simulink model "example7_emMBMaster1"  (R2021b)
settings: Solver=FixedStepAuto  StartTime=0  StopTime=inf  FixedStep=0.5  RelTol=1e-3  EnableMultiTasking=on
undefined symbols (not defined in the file or in its folder): based, classic, Coils, Discretes, dsPic33, InputsReg, MCC, Microchip, PIC24, Read
libraries: emMBMastedLib x8, embeddedCreatorLib x1

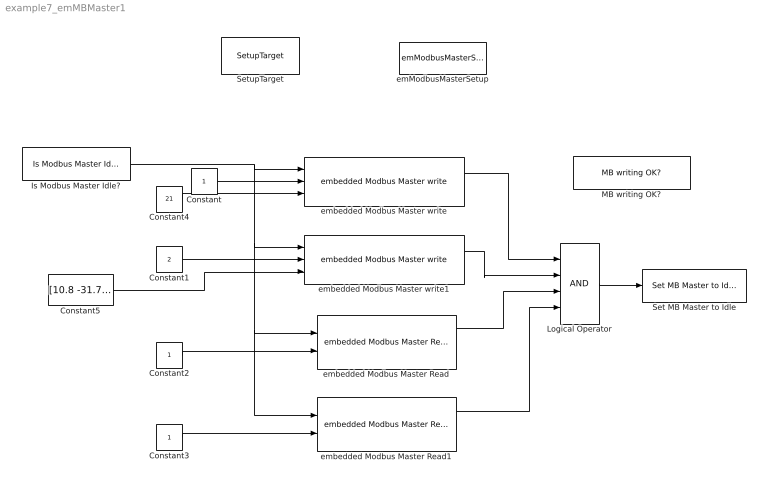
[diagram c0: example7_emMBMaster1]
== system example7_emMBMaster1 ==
  Constant : Constant  OutDataTypeStr=uint16
  Constant1 : Constant  Value=2  OutDataTypeStr=uint16
  Constant2 : Constant  OutDataTypeStr=uint16
  Constant3 : Constant  OutDataTypeStr=uint16
  Constant4 : Constant  Value=21  OutDataTypeStr=uint16
  Constant5 : Constant  Value=[10.8 -31.77]  OutDataTypeStr=single
  Is Modbus Master Idle? : emMBMastedLib/Is Modbus Master Idle?  Tag=isMB_Idle  c_sampleTime=-1
  Logical Operator : Logic  Inputs=4  AllPortsSameDT=off  OutDataTypeStr=boolean
  MB writing OK? : emMBMastedLib/MB writing OK?  c_writeNo=1  c_sampleTime=-1
  Set MB Master to Idle : emMBMastedLib/Set MB Master to Idle  Tag=setMB2Idle
  SetupTarget : embeddedCreatorLib/SetupTarget  Tag=SetupTarget  Priority=0  c_platform=Microchip PIC24/dsPic33 based on MCC classic  c_debug=on
  emModbusMasterSetup : emMBMastedLib/emModbusMasterSetup  Tag=emModbusMasterSetup  c_uartNo=1  c_baudrate=19200  c_forceLongerSpace=on  c_writeServerID="[2  4 7 ]"  c_writeCMD1Type=Single-Write-holding  c_writeCMD2Type=Multiple-Write-holdings  c_writeCMD3Type=Multiple-Write-coils  c_writeCMD4Type=Single-Write-holding  c_writeCMD5Type=Single-Write-holding  c_writeCMD6Type=Single-Write-holding  c_writeCMD7Type=Single-Write-holding  c_writeCMD8Type=Single-Write-holding  c_writeCMD9Type=Single-Write-holding  c_writeCMD10Type=Single-Write-holding  c_writeCMD11Type=Single-Write-holding  c_writeCMD12Type=Single-Write-holding  c_writeCMD13Type=Single-Write-holding  c_writeCMD14Type=Single-Write-holding  c_writeCMD15Type=Single-Write-holding  c_writeRegMAXQTY=[1 8 45]  c_readCMD1Type=Read-InputsReg  c_readCMD2Type=Read-Discretes  c_readCMD3Type=Read-Coils  c_readCMD4Type=Read-Discretes  c_readCMD5Type=Read-InputsReg  c_readCMD6Type=Read-InputsReg  c_readCMD7Type=Read-InputsReg  c_readCMD8Type=Read-InputsReg  c_readCMD9Type=Read-InputsReg  c_readCMD10Type=Read-InputsReg  c_readCMD11Type=Read-InputsReg  c_readCMD12Type=Read-InputsReg  c_readCMD13Type=Read-InputsReg  c_readCMD14Type=Read-InputsReg  c_readCMD15Type=Read-InputsReg  c_readCMD16Type=Read-InputsReg  c_readRegMAXQTY=[30 7 200 300 5 6 7 8 9 10 11 12 13 14 15]  c_MaxTry=10  c_Timeout=800  c_Name_method=By phycical port name and bit number  c_PortName=B  c_BitNo=2  c_txEnable485="\"LATBbits.LATB2\""  c_TxEnable485Polarity=on
  embedded Modbus Master Read : emMBMastedLib/embedded Modbus Master Read  Tag=ModbusMasterReading  c_SeverID=1  c_readNo=1  c_dataType=Unsigned 32 bits int  c_dataQTY=2  c_endian=Big-endian
  embedded Modbus Master Read1 : emMBMastedLib/embedded Modbus Master Read  Tag=ModbusMasterReading  c_SeverID=2  c_readNo=2  c_dataType=Logical boolean  c_dataQTY=7  c_endian=Big-endian
  embedded Modbus Master write : emMBMastedLib/embedded Modbus Master write  Tag=ModbusMasterWriting  c_SeverID=[1 2]  c_writeNo=1  c_endian=Big-endian
  embedded Modbus Master write1 : emMBMastedLib/embedded Modbus Master write  Tag=ModbusMasterWriting  c_SeverID=[3 4]  c_writeNo=2  c_endian=Big-endian
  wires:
  Is Modbus Master Idle?/1 -> embedded Modbus Master write/1, embedded Modbus Master write1/1, embedded Modbus Master Read1/1, embedded Modbus Master Read/1
  Constant/1 -> embedded Modbus Master write/2
  Constant4/1 -> embedded Modbus Master write/3
  Constant5/1 -> embedded Modbus Master write1/3
  Constant1/1 -> embedded Modbus Master write1/2
  Constant2/1 -> embedded Modbus Master Read/2
  Constant3/1 -> embedded Modbus Master Read1/2
  embedded Modbus Master write/1 -> Logical Operator/1
  embedded Modbus Master write1/1 -> Logical Operator/2
  embedded Modbus Master Read/1 -> Logical Operator/3
  embedded Modbus Master Read1/1 -> Logical Operator/4
  Logical Operator/1 -> Set MB Master to Idle/1
